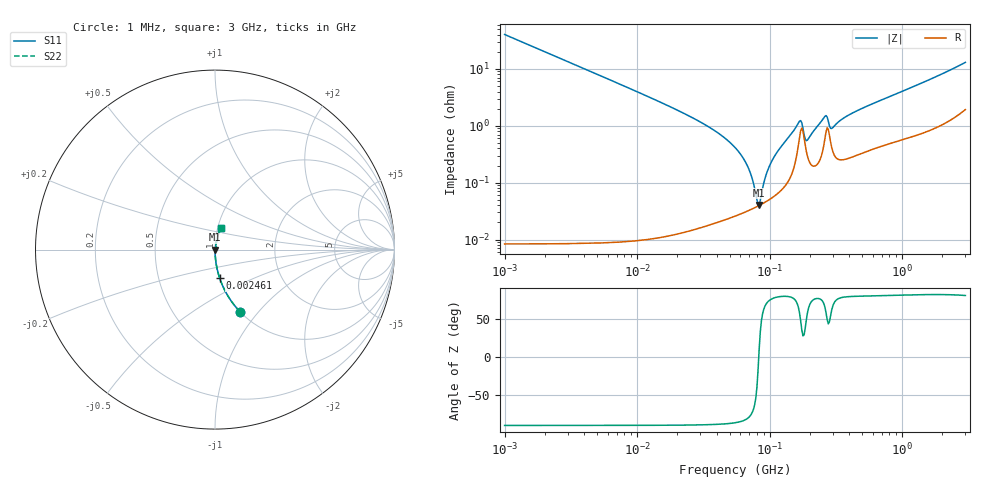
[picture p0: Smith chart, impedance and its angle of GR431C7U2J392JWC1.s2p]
!Murata Part Number: GR431C7U2J392JWC1
!These Parameters are Measured in Series Mode Connection
!Data Generated on Jun 10, 2025
!  o--ll--o
!Port1  Port2
!  o------o
!Operation Temp=25[degC], DC Bias Voltage=0[V]
!Freq. Start=1000[kHz] Stop=3[GHz] 401[Steps]
# Hz S RI R 50
!Freq.(Hz) S11(Real) S11(Imag) S21(Real) S21(Imag) S12(Real) S12(Imag) S22(Real) S22(Imag)
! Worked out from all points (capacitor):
!   401 points, 1 MHz to 3 GHz, reference 50 ohm
!   read as one part in series: C = 3.96 nF near 1.041 MHz
!   lowest |Z| = 40.5 mohm at 83.39 MHz (marker M1)
!   series resonance near 82.74 MHz, so ESL is about 940 pH
!   S11 on the Smith chart (normalised r, x): 1 MHz: 1.00, -0.80; 2.461 MHz: 1.00, -0.33; 3 GHz: 1.04, +0.26
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1000000  0.1394 -0.3462  0.8606 0.3462  0.8606 0.3462  0.1394 -0.3462
2461366  0.0261 -0.1591  0.9739 0.1591  0.9739 0.1591  0.0261 -0.1591
3823119  0.011 -0.1039  0.989 0.1039  0.989 0.1039  0.011 -0.1039
1.461624e7  0.000817 -0.0266  0.9992 0.0266  0.9992 0.0266  0.000817 -0.0266
3.387922e7  0.000273 -0.00988  0.9997 0.00988  0.9997 0.00988  0.000273 -0.00988
5.477226e7  0.000275 -0.00414  0.9997 0.00414  0.9997 0.00414  0.000275 -0.00414
6.826239e7  0.000321 -0.0019  0.9997 0.0019  0.9997 0.0019  0.000321 -0.0019
7.395247e7  0.000347 -0.00111  0.9997 0.00111  0.9997 0.00111  0.000347 -0.00111
8.011685e7  0.000378 -0.000319  0.9996 0.000319  0.9996 0.000319  0.000378 -0.000319
8.338914e7  0.000397 7.8e-05  0.9996 -7.8e-05  0.9996 -7.8e-05  0.000397 7.8e-05
9.402997e7  0.000465 0.00129  0.9995 -0.00129  0.9995 -0.00129  0.000465 0.00129
1.039275e8  0.000544 0.00235  0.9995 -0.00235  0.9995 -0.00235  0.000544 0.00235
1.646891e8  0.00463 0.0102  0.9954 -0.0102  0.9954 -0.0102  0.00463 0.0102
1.714156e8  0.00824 0.00904  0.9918 -0.00904  0.9918 -0.00904  0.00824 0.00904
1.894586e8  0.0035 0.00417  0.9965 -0.00417  0.9965 -0.00417  0.0035 0.00417
2.094008e8  0.00204 0.00717  0.998 -0.00717  0.998 -0.00717  0.00204 0.00717
2.609752e8  0.00598 0.0132  0.994 -0.0132  0.994 -0.0132  0.00598 0.0132
2.884452e8  0.00518 0.00729  0.9948 -0.00729  0.9948 -0.00729  0.00518 0.00729
3.002264e8  0.00354 0.00859  0.9965 -0.00859  0.9965 -0.00859  0.00354 0.00859
4.0536e8  0.00297 0.0156  0.997 -0.0156  0.997 -0.0156  0.00297 0.0156
8.005644e8  0.00582 0.0317  0.9942 -0.0317  0.9942 -0.0317  0.00582 0.0317
3e9  0.0343 0.122  0.9657 -0.122  0.9657 -0.122  0.0343 0.122
